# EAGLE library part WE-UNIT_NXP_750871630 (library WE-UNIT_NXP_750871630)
Off-Line Transformer WE-Unit NXP - Nominal input voltage: 85-265 VAC - Operating temperature: -40°C to +125 °C - Isolation voltage 4 kVAC -- Especially designed for several ICs from NXP TEA1623PH -- Universal input -- Smart meters -- Dimmable 12 V LED driver -- Offline-switch mode power supplies
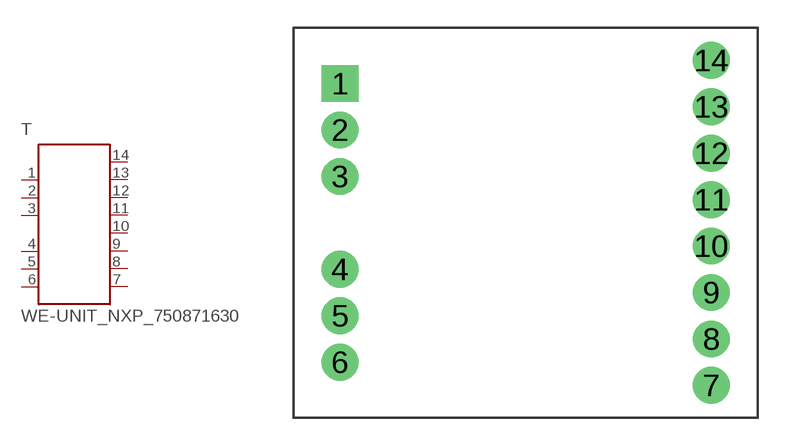
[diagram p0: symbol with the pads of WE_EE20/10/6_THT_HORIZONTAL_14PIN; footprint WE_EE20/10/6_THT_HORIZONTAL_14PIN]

Designator prefix T

## WE-UNIT_NXP_750871630 (MPN: 750871630; OC_FARNELL: 1849057; OC_NEWARK: 13T9846; PACKAGE: EE20_10_6_NXP; SUPPLIER: Würth Elektronik eiSos GmbH)  [WE_EE20/10/6_THT_HORIZONTAL_14PIN]
1  1  pas
2  2  pas
3  3  pas
4  4  pas
5  5  pas
6  6  pas
7  7  pas
8  8  pas
9  9  pas
10  10  pas
11  11  pas
12  12  pas
13  13  pas
14  14  pas

## Footprint WE_EE20/10/6_THT_HORIZONTAL_14PIN (pad centres in mm)
Transformer, EE20/10/6 THT Horizontal 14 Pin
drill 1.32 square: 1 -10,7.5
drill 1.32: 2 -10,5; 3 -10,2.5; 4 -10,-2.5; 5 -10,-5; 6 -10,-7.5; 7 10,-8.75; 8 10,-6.25; 9 10,-3.75; 10 10,-1.25; 11 10,1.25; 12 10,3.75; 13 10,6.25; 14 10,8.75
